(* Logix 5000 AddOnInstructionDefinition export MAH_Yaskawa; software revision 17.00 *)

TYPE Yaskawa_EIP_Servo :   // Yaskawa SigmaLogic Axis Structure v2.4.0
STRUCT
   O : Yaskawa_OUT_to_Servo;
   I : Yaskawa_IN_from_Servo;
   AOI_SB : Yaskawa_AOI_Status_Bits;
END_STRUCT
END_TYPE

TYPE Yaskawa_OUT_to_Servo :   // Structure of data sent out to the Yaskawa SigmaLogic controller v2.4.0
STRUCT
   b00_ServoOn : BOOL;   // Servo On
   b01_Stop : BOOL;   // Stops All Current Motion in Progress
   b02_Home : BOOL;   // Start Homing Process
   b03_MoveStart1 : BOOL;   // Start Current Motion
   b06_SuperImpose : BOOL;
   b07_ServoAlarmReset : BOOL;   // Servo Alarm Reset
   b08_ControllerAlarmReset : BOOL;   // SigmaLogic Alarm Reset
   b09_MoveStart2 : BOOL;   // Start Second Motion (Blended Move)
   b10_MoveAbort : BOOL;   // Abort Current Move
   b11_MovePause : BOOL;   // Pause Current Move
   b12_SeqPause : BOOL;   // Indexing Sequence Pause
   b13_SeqResume : BOOL;   // Indexing Sequence Resume
   b14_SeqCancel : BOOL;   // Indexing Sequence Cancel
   b15_AbsEncoderReset : BOOL;   // Absolute Encoder Reset
   b16_SeqStart : BOOL;   // Start Indexing Sequence
   b17_SeqEditSpeed : BOOL;   // Enter Edit Speed
   b18_SeqEditDistance : BOOL;   // Enter Distance Edit
   b19_PLSEnable : BOOL;   // Enable PLS execution
   b20_PLSActivateOutput1 : BOOL;   // Activate PLS output1 switch logic
   b21_PLSActivateOutput2 : BOOL;   // Activate PLS output2 switch logic
   b22_PLSActivateOutput3 : BOOL;   // Activate PLS output3 switch logic
   b23_PLSActivateOutput4 : BOOL;   // Activate PLS output4 switch logic
   b24_SetClock : BOOL;   // Set the remote controller clock with data provided by the PLC
   RebootController : BOOL;
   UseExternalEncoder : BOOL;   // Use External Encoder when executing MAHSP_Yaskawa
   b32_HeatbeatAnswer : BOOL;   // Heartbeat Answer
   BrakeBypassRequest : BOOL;
   SetFwdTorqueLimit : BOOL;
   SetRevTorqueLimit : BOOL;
   TorqueLimit : DINT;
   TorqueRamp : DINT;
   HomeMethod : INT;
   HomeSpeed : DINT;
   HomeAccDec : DINT;   // Home Move Acceleration/Deceleration Rate
   HomeBackOffDistance : DINT;
   HomeCreepSpeed : DINT;
   HomeCreepDistanceLimit : DINT;
   HomeCreepTimeLimit : DINT;
   HomeOffsetDistance : DINT;
   HomeOffsetSpeed : DINT;
   HomePostion : DINT;
   HomeTorque : DINT;
   HomeInputNo : DINT;
   HomeApproachTimeLimit : DINT;
   HomeApproachDistLimit : DINT;
   HomeDirection : INT;
   HomeSwitchMode : INT;
   MoveType : INT;
   MoveDirection : INT;
   MoveAccel1 : DINT;
   MoveAccel2 : DINT;
   MoveDecel1 : DINT;
   MoveDecel2 : DINT;
   MoveSpeed1 : DINT;
   MoveSpeed2 : DINT;
   MoveDistance1 : DINT;
   MoveDistance2 : DINT;
   MovePosition1 : DINT;
   MovePosition2 : DINT;
   RegistrationDistance : DINT;
   GearNumerator : DINT;
   GearDenominator : DINT;
   SuperImposeDistance : DINT;
   Resolution : INT;
   RegistrationDirection : INT;
   TuningLevel : INT;
   SequenceStep : INT;   // Staring Sequence Step Number
   SequenceEditStep : INT;   // Sequence Step Number to Edit
   FlagCommandBits1 : DINT;   // Flag Commands. 1..64 are General Flags, Bits 0..31 correspond to Flag 1..32
   FlagCommandBits2 : DINT;   // Flag Commands cont. 1..64 are General Flags, Bits 0..31 correspond to Flag 33..64
   DigitalOutCommandBits : DINT;   // Digital Output commands. Bits 0-7 correspond to CN13 Digital Outputs 0-7, used as Flag 73-80. Bits 8-10 correspond to CN1 Digital Outputs 0-2 used as Flag 88-90"
   SequenceEditSpeed : DINT;
   SequenceEditDistance : DINT;
   FeedRateOverride : INT;
   HSI_Enable : BOOL;
   HSI_MoveMode : BOOL;   // 0=Relative; 1=Moves per Cycle
   HSI_CalcMethod : BOOL;   // 0=Accel/Decel; 1=Time
   HSI_MoveDirection : BOOL;   // 0 = Negative; 1 = Positive
   HSI_TriggerFlag : INT;
   HSI_MovingFlag : INT;
   HSI_DwellingFlag : INT;
   HSI_DoneFlag : INT;
   HSI_MoveType : INT;   // 0=Single; 1=Repeat; 2=Repeat "x" times
   HSI_RepeatNumber : INT;
   HSI_Distance : DINT;
   HSI_Speed : DINT;
   HSI_Accel : DINT;
   HSI_MoveTime : DINT;
   HSI_DwellTime : DINT;
   PLS_OutputFlag1 : INT;
   PLS_OutputFlag2 : INT;
   PLS_OutputFlag3 : INT;
   PLS_OutputFlag4 : INT;
   PLS_OnPosition1 : DINT;
   PLS_OffPosition1 : DINT;
   PLS_OnPosition2 : DINT;
   PLS_OffPosition2 : DINT;
   PLS_OnPosition3 : DINT;
   PLS_OffPosition3 : DINT;
   PLS_OnPosition4 : DINT;
   PLS_OffPosition4 : DINT;
   PLS_OnCompensation1 : INT;
   PLS_OffCompensation1 : INT;
   PLS_OnCompensation2 : INT;
   PLS_OffCompensation2 : INT;
   PLS_OnCompensation3 : INT;
   PLS_OffCompensation3 : INT;
   PLS_OnCompensation4 : INT;
   PLS_OffCompensation4 : INT;
   RTC_Year : INT;
   RTC_Month : INT;
   RTC_Day : INT;
   RTC_Hour : INT;
   RTC_Min : INT;
   RTC_Sec : INT;
   StopDecel : DINT;
   AnalogOutput : INT;   // CN13, AO_01 [mV]
END_STRUCT
END_TYPE

TYPE Yaskawa_AOI_Status_Bits :   // Internal bits used to interlock Yaskawa AOI execution. v2.4.0
STRUCT
   MAM : BOOL;   // Move AOI Active
   MAJ : BOOL;   // Jog AOI Active
   MAB : BOOL;   // Blending AOI Active
   MAG : BOOL;   // Gearing AOI Active
   MAHSP : BOOL;   // Home SetPoint AOI Active
   MAH : BOOL;   // Homing AOI Active
   MSQE : BOOL;   // Sequence Edit AOI Active
   MSQR : BOOL;   // Sequence Run AOI Active
   MHSI : BOOL;   // High Speed Index AOI Active
   MSO : BOOL;   // Servo On
   MSF : BOOL;   // Servo Off
   MAFR : BOOL;   // Fault Reset
   MAS : BOOL;   // Servo Abort
   MTRQ : BOOL;   // Torque Mode Active
   MPLS : BOOL;   // PLS Active
   MCLK : BOOL;   // SetClock Active
   MSTL : BOOL;   // Set Torque Limit Active
   AOI_Permissive : BOOL;   // Permissive to Execute an AOI
END_STRUCT
END_TYPE

TYPE Yaskawa_IN_from_Servo :   // Structure of data coming from the Yaskawa SigmaLogic controller. v2.4.0
STRUCT
   AlarmText : STRING;   // ServoPack Alarm Code plus Text Description
   b00_Heartbeat : BOOL;
   b01_Alarm : BOOL;   // ServoPack Alarm
   b02_Warning : BOOL;   // ServoPack Warning
   b03_Ready : BOOL;   // ServoPack Ready
   b04_Enabled : BOOL;   // ServoPack Enabled ("Servo On")
   b05_StopComplete : BOOL;
   b06_HomeComplete : BOOL;
   b07_HomeBusy : BOOL;
   b08_HomeActive : BOOL;
   b09_HomeAborted : BOOL;
   b10_HomeError : BOOL;
   b11_MoveAbsComplete : BOOL;
   b12_MoveAbsBusy : BOOL;
   b13_MoveAbsActive : BOOL;
   b14_MoveAbsAborted : BOOL;
   b15_MoveAbsError : BOOL;
   b16_MoveRelComplete : BOOL;
   b17_MoveRelBusy : BOOL;
   b18_MoveRelActive : BOOL;
   b19_MoveRelAborted : BOOL;
   b20_MoveRelError : BOOL;
   b21_JogAtSpeed : BOOL;
   b22_JogBusy : BOOL;
   b23_JogActive : BOOL;
   b24_JogAborted : BOOL;
   b25_JogError : BOOL;
   b26_GearInSync : BOOL;
   b27_GearBusy : BOOL;
   b28_GearActive : BOOL;
   b29_GearAborted : BOOL;
   b30_GearError : BOOL;
   b32_MoveSuperComplete : BOOL;
   b33_MoveSuperBusy : BOOL;
   b34_MoveSuperActive : BOOL;
   b35_MoveSuperAborted : BOOL;
   b36_MoveSuperError : BOOL;
   b37_PowerCycleRequired : BOOL;
   b38_MoveBlend1Complete : BOOL;
   b39_MoveBlend1Busy : BOOL;
   b40_MoveBlend1Active : BOOL;
   b41_MoveBlend1Abort : BOOL;
   b42_MoveBlend1Error : BOOL;
   b43_MoveBlend2Complete : BOOL;
   b44_MoveBlend2Busy : BOOL;
   b45_MoveBlend2Active : BOOL;
   b46_MoveBlend2Abort : BOOL;
   b47_MoveBlend2Error : BOOL;
   b48_RegComplete : BOOL;
   b49_RegBusy : BOOL;
   b50_RegActive : BOOL;
   b51_RegAborted : BOOL;
   b52_RegError : BOOL;
   b53_ResetAbsEncoderActive : BOOL;
   b54_ResetAbsEncoderBusy : BOOL;
   b55_ResetAbsEncoderDone : BOOL;
   b56_ResetAbsEncoderError : BOOL;
   b57_SeqRunning : BOOL;
   b58_RegSensorNotReached : BOOL;
   b59_SeqEditError : BOOL;
   b60_SeqEditDone : BOOL;
   b61_TorqueAtTorque : BOOL;
   b62_TorqueBusy : BOOL;
   b63_TorqueActive : BOOL;
   b64_TorqueAborted : BOOL;
   b65_TorqueError : BOOL;
   b66_ControllerAlarm : BOOL;
   b67_ApplicationError : BOOL;
   b68_AxisAtStandStill : BOOL;
   b69_TestModeActive : BOOL;
   b70_ServoParamsOK : BOOL;
   b71_SetFwdTorqueLimitDone : BOOL;
   b72_SetRevTorqueLimitDone : BOOL;
   Position : DINT;
   Speed : DINT;
   Torque : DINT;
   HomeErrorID : INT;
   MoveAbsErrorID : INT;
   MoveRelErrorID : INT;
   JogErrorID : INT;
   GearErrorID : INT;
   MoveSuperErrorID : INT;
   ServoAlarmID : INT;
   ServoWarningID : INT;
   ControllerAlarmID : DINT;
   AxisGenAlarmID : DINT;
   MoveBlend1ErrorID : INT;
   MoveBlend2ErrorID : INT;
   ResetAbsEncoderErrorID : INT;
   FunctionBlockErrorID : INT;
   TorqueErrorID : INT;
   RegErrorID : INT;
   SeqCurrentStep : INT;
   FlagStatusBit1 : DINT;   // Flag Status. 1..64 are General Flags, Bits 0..31 correspond to Flag 1..32
   FlagStatusBit2 : DINT;   // Flag Status cont. 1..64 are General Flags, Bits 0..31 correspond to Flag 33..64
   IOStatusBits : DINT;   // Digital IO Status. Bits 0-7, CN13 Inputs 0-7, Used as Flag 65-72. Bits 8-15, CN13 Outputs 0-7, Used as Flag 73-80. Bits 16-22, CN1 Inputs 0-6, Used as Flag 81-87. Bits 23-25, CN1 Outputs 0-4, Used as Flag 88-92.
   HSI_Moving : BOOL;
   HSI_Dwelling : BOOL;
   HSI_Done : BOOL;
   HSI_Busy : BOOL;
   HSI_Error : BOOL;
   HSI_ErrorCode : INT;
   PLS_Running : BOOL;
   PLS_SwitchStatus1 : BOOL;
   PLS_SwitchStatus2 : BOOL;
   PLS_SwitchStatus3 : BOOL;
   PLS_SwitchStatus4 : BOOL;
   PLS_Busy : BOOL;
   PLS_Error : BOOL;
   PLS_ErrorCode : INT;
   SetClock_Done : BOOL;
   SetClock_Busy : BOOL;
   SetClock_Error : BOOL;
   SetClock_ErrorID : INT;
   SoftwareVersion : DINT;
   FirmwareVersion : DINT;
   CommandedPos : DINT;
   CommandedPosNonCyc : DINT;
   CommandedSpeed : DINT;
   Clock_Year : INT;
   Clock_Month : INT;
   Clock_Day : INT;
   Clock_Hour : INT;
   Clock_Minute : INT;
   Clock_Second : INT;
   AnalogInput : REAL;   // CN13, AI_01 [v]
   BrakeBypassActive : BOOL;
   ForwardTorqueLimit : DINT;
   ReverseTorqueLimit : DINT;
END_STRUCT
END_TYPE

ADD_ON_INSTRUCTION MAH_Yaskawa   (* revision 2.4 0, vendor Yaskawa America, Inc., ExecuteEnableInFalse *)
// Motion Axis Home
// Revision note:
// 2.4.0: Improved Error Codes for invalid homing parameters.
// 2.3.1: Moved unlatch of AOI_ON_LOCAL to bottom of EnableInFalse routine so that outputs will be on for at least 1 scan if one-shot on EN is used.
// 2.3.0: No functional change
// 2.0.0: Added new Homing type for C-Pulse Only (Type 4), The ORDER OF THE INPUTS HAS CHANGED. Check attached tags for existing projects!
// Help:
// This AOI moves a servo axis to a home position by various methods. Timeouts are not directly included in this AOI and should be implemented in user code. Supported Homing Methods include:
// - Set Position Only
// - To Hard Stop.
// - To Overtravel (P-OT, N-OT) w/wo encoder C-Channel
// - To Flag w/wo encoder C-Channel (Flag can also be one of the Controller Digital Inputs)
//     CN1 Inputs: SI0...SI6 = Flag 81...Flag 87
//     CN13 Inputs: DI_00... DI_07 = Flag 65...Flag72
// 'Set Position Only' can occur whether the servo is enabled or disabled. Position will be immediately set to the specified value.
// Home to Hard Stop moves the servo under a Torque Limit until the hard stop is reached according to the following sequence:
// - Backoff move is always performed in the opposite direction of the search Direction. Always use a Positive Value for BackoffDistance
// - TorqueLimit is set and the axis moves to the hard stop in the specified Direction under max Speed limit.
// - When hard stop is reached, Offset move is performed according to the value set in OffsetDistance and OffsetSpeed. Direction will always be opposite to the searching direction.
// - Position is defined as the SetPosition
// Home to Overtravel (P-OT, N-OT) or Flag without C-Channel performs the following sequence:
// - Initial search (Approach) in specified Direction.
// - TorqueLimit is active
// - When Overtravel switch or Flag is found,  move the BackoffDistance. Always use a Positive Value for BackoffDistance. Direction will be automatically opposite of search direction
// - Final search is performed (Creep) in the specified Direction using CreepSpeed
// - When Overtravel switch or Flag is found again,  Offset move is performed according to the value set in OffsetDistance and OffsetSpeed. Direction will be automatically opposite of serach direction.
// - Position is defined as the SetPosition
// Home to Overtravel (P-OT, N-OT) or Flag with C-Channel performs the following sequence:
// - Initial search (Approach) in specified Direction.
// - TorqueLimit is active
// - When Overtravel switch or Flag is found,  move the BackoffDistance. Always use a Positive Value for BackoffDistance. Direction will be automatically opposite of search direction
// - Final search is performed (Creep) in the specified Direction using CreepSpeed
// - When C-Channel is found,  Offset move is performed according to the value set in OffsetDistance and OffsetSpeed. Direction will be automatically opposite of serach direction.
// - Position is defined as the SetPosition
// Error Codes:
// 13017: Invalid Homing Parameters
// 13018: Invalid Move Type - Overtravel(s) are disabled
// 13019: Home Input not found
// 13020: Invalid Homing Type
// 13021: Invalid Accel/Decel Parameter
// 13022: Invalid Velocity Parameter
// 13023: Invalid Torque Parameter
// 13024: Invalid Position Parameter
VAR_IN_OUT
   Axis : Yaskawa_EIP_Servo; {required}
END_VAR
VAR_INPUT
   HomeType : INT := 1; {required}   // 0 = Set Position 1 = Home to Hard Stop 2 = Home to Overtravel Switch 3 = Home to Flag 4= Home to C-Pulse Only
   Direction : INT; {required}   // 0 = Positive 1 = Negative
   Use_CPulse : INT; {required}   // 0 = Do Not Use C-Pulse 1 = Use C-Pulse
   Accel_Decel : REAL; {required}   // Homing Accel/Decel [unit/s/s]
   Speed : REAL; {required}   // Homing Speed [unit/s]
   TorqueLimit : REAL; {required}   // Torque or Force Limit for Homing [%motor rated torque/force]
   FlagNo : INT; {required}   // SigmaLogic Flag to use as Trigger for Home Type 3
   BackoffDistance : REAL; {required}   // Distance to back off before moving to hard stop (Type 1) or after finding the overtravel or flag (Types 2 and 3)
   CreepSpeed : REAL; {required}   // Homing Creep Speed [units/s]
   OffsetDistance : REAL; {required}   // Homing Offset Distance [unit]
   OffsetSpeed : REAL; {required}   // Homing Offset Speed [unit/s]
   SetPosition : REAL; {required}   // Position to Define at end of homing process
   ApproachDistanceLimit : REAL;   // (Not supported)
   ApproachTimeLimit : REAL;   // (Not supported)
   CreepDistLimit : REAL;   // (Not supported)
   CreepTimeLimit : REAL;   // (Not supported)
END_VAR
VAR_OUTPUT
   EN : BOOL; {visible}   // The AOI is Active
   DN : BOOL; {visible}   // Homing is Done
   IP : BOOL; {visible}   // Homing is In Process
   ER : BOOL; {visible}   // Homing Process Error
   PC : BOOL; {visible}   // Homing Process is Successfully Completed
   FLT_RDY : BOOL; {visible}   // The Servo is Not Ready
   FLT_BSY : BOOL; {visible}   // There is another AOI Active for this Axis
   ErrorCode : INT; {visible}   // Homing process Error Code
END_VAR
VAR
   AOI_ON_LOCAL : BOOL;
   ScaleFactor : DINT;
   Finished : BOOL;   // Function is finished
   Execute_OS : BOOL;
END_VAR

ROUTINE EnableInFalse   (* ladder *)
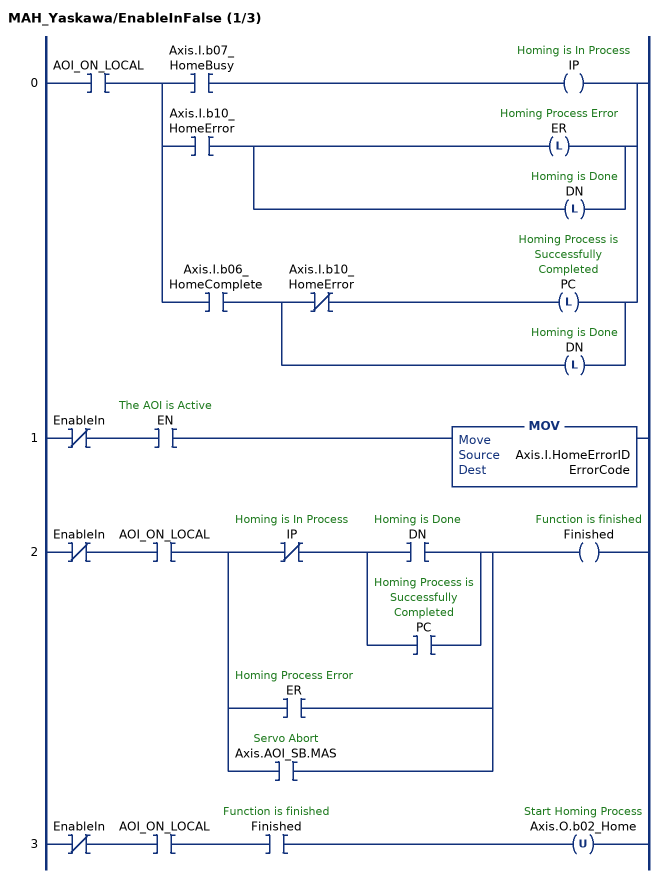
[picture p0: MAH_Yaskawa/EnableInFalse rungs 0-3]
   0: XIC(AOI_ON_LOCAL)[XIC(Axis.I.b07_HomeBusy) OTE(IP) ,XIC(Axis.I.b10_HomeError) [OTL(ER) ,OTL(DN) ] ,XIC(Axis.I.b06_HomeComplete) [XIO(Axis.I.b10_HomeError) OTL(PC) ,OTL(DN) ] ];
   1: XIO(EnableIn)XIC(EN)MOV(Axis.I.HomeErrorID,ErrorCode);
   2: XIO(EnableIn)XIC(AOI_ON_LOCAL)[XIO(IP) [XIC(DN) ,XIC(PC) ] ,XIC(ER) ,XIC(Axis.AOI_SB.MAS) ]OTE(Finished);
   3: XIO(EnableIn)XIC(AOI_ON_LOCAL)XIC(Finished)OTU(Axis.O.b02_Home);
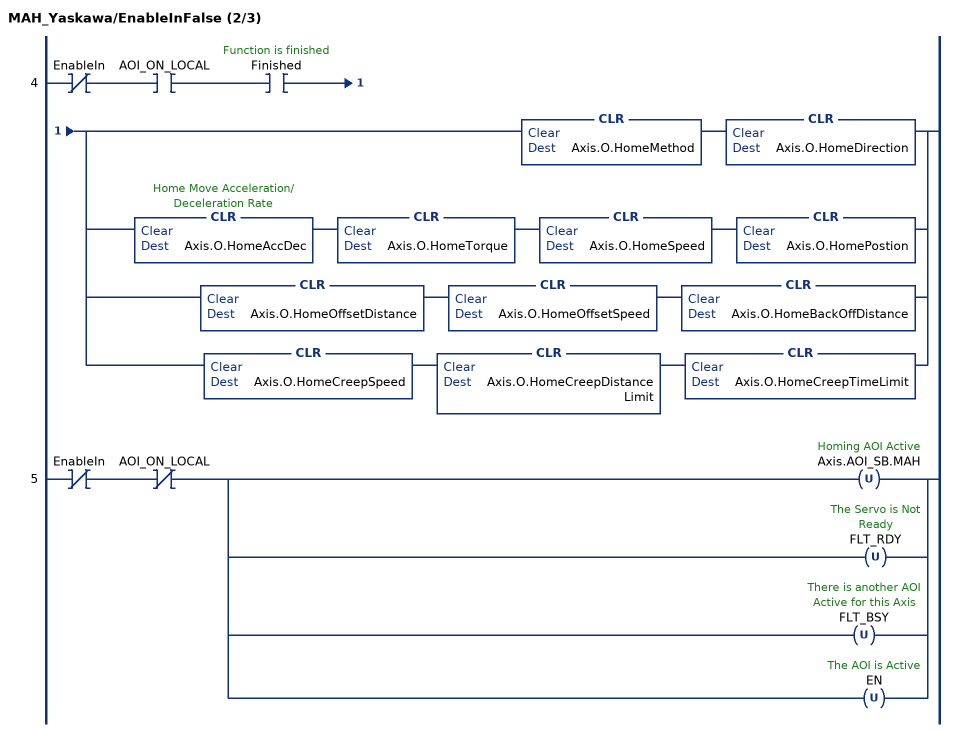
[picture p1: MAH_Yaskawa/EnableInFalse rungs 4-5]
   4: XIO(EnableIn)XIC(AOI_ON_LOCAL)XIC(Finished)[CLR(Axis.O.HomeMethod) CLR(Axis.O.HomeDirection) ,CLR(Axis.O.HomeAccDec) CLR(Axis.O.HomeTorque) CLR(Axis.O.HomeSpeed) CLR(Axis.O.HomePostion) ,CLR(Axis.O.HomeOffsetDistance) CLR(Axis.O.HomeOffsetSpeed) CLR(Axis.O.HomeBackOffDistance) ,CLR(Axis.O.HomeCreepSpeed) CLR(Axis.O.HomeCreepDistanceLimit) CLR(Axis.O.HomeCreepTimeLimit) ];
   5: XIO(EnableIn)XIO(AOI_ON_LOCAL)[OTU(Axis.AOI_SB.MAH) ,OTU(FLT_RDY) ,OTU(FLT_BSY) ,OTU(EN) ];
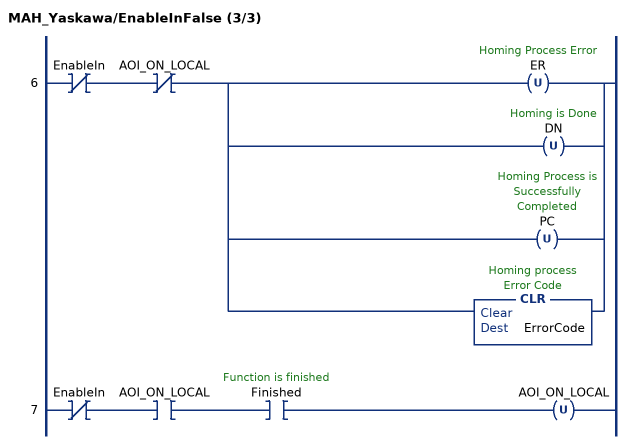
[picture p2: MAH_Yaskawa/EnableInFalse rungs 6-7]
   6: XIO(EnableIn)XIO(AOI_ON_LOCAL)[OTU(ER) ,OTU(DN) ,OTU(PC) ,CLR(ErrorCode) ];
   7: XIO(EnableIn)XIC(AOI_ON_LOCAL)XIC(Finished)OTU(AOI_ON_LOCAL);
END_ROUTINE

ROUTINE Logic   (* ladder *)
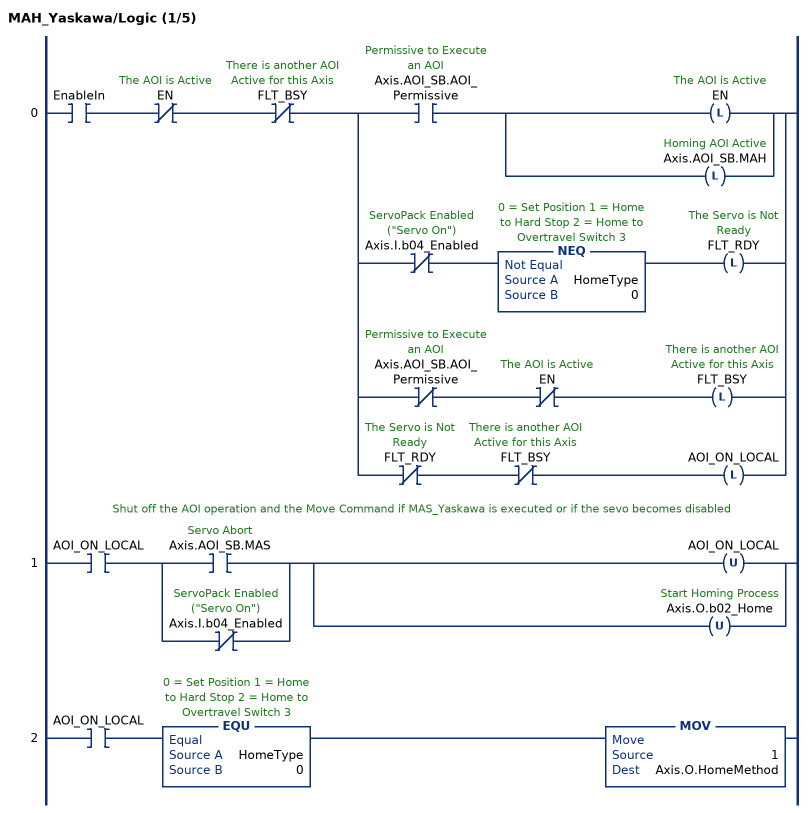
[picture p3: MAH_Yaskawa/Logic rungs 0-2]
   0: XIC(EnableIn)XIO(EN)XIO(FLT_BSY)[XIC(Axis.AOI_SB.AOI_Permissive) [OTL(EN) ,OTL(Axis.AOI_SB.MAH) ] ,XIO(Axis.I.b04_Enabled) NEQ(HomeType,0) OTL(FLT_RDY) ,XIO(Axis.AOI_SB.AOI_Permissive) XIO(EN) OTL(FLT_BSY) ,XIO(FLT_RDY) XIO(FLT_BSY) OTL(AOI_ON_LOCAL) ];
   // Shut off the AOI operation and the Move Command if MAS_Yaskawa is executed or if the sevo becomes disabled
   1: XIC(AOI_ON_LOCAL)[XIC(Axis.AOI_SB.MAS) ,XIO(Axis.I.b04_Enabled) ][OTU(AOI_ON_LOCAL) ,OTU(Axis.O.b02_Home) ];
   2: XIC(AOI_ON_LOCAL)EQU(HomeType,0)MOV(1,Axis.O.HomeMethod);
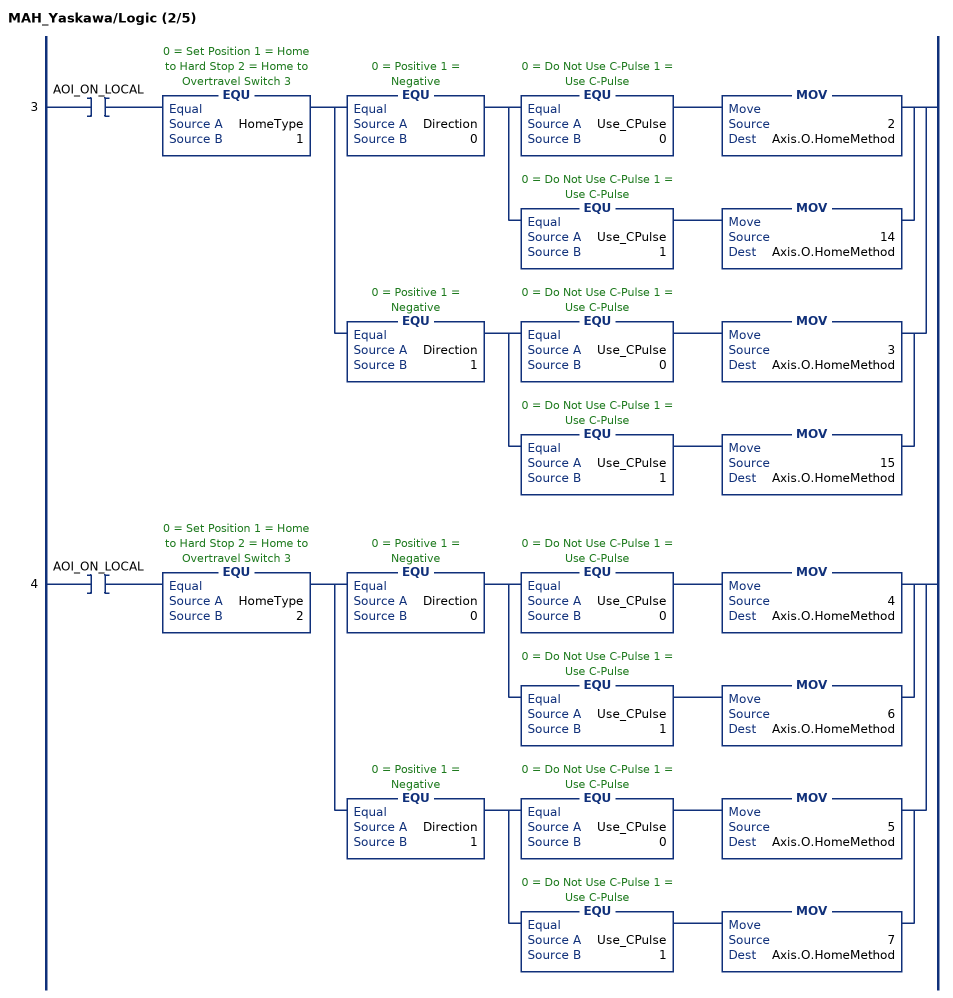
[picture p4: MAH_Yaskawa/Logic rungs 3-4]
   3: XIC(AOI_ON_LOCAL)EQU(HomeType,1)[EQU(Direction,0) [EQU(Use_CPulse,0) MOV(2,Axis.O.HomeMethod) ,EQU(Use_CPulse,1) MOV(14,Axis.O.HomeMethod) ] ,EQU(Direction,1) [EQU(Use_CPulse,0) MOV(3,Axis.O.HomeMethod) ,EQU(Use_CPulse,1) MOV(15,Axis.O.HomeMethod) ] ];
   4: XIC(AOI_ON_LOCAL)EQU(HomeType,2)[EQU(Direction,0) [EQU(Use_CPulse,0) MOV(4,Axis.O.HomeMethod) ,EQU(Use_CPulse,1) MOV(6,Axis.O.HomeMethod) ] ,EQU(Direction,1) [EQU(Use_CPulse,0) MOV(5,Axis.O.HomeMethod) ,EQU(Use_CPulse,1) MOV(7,Axis.O.HomeMethod) ] ];
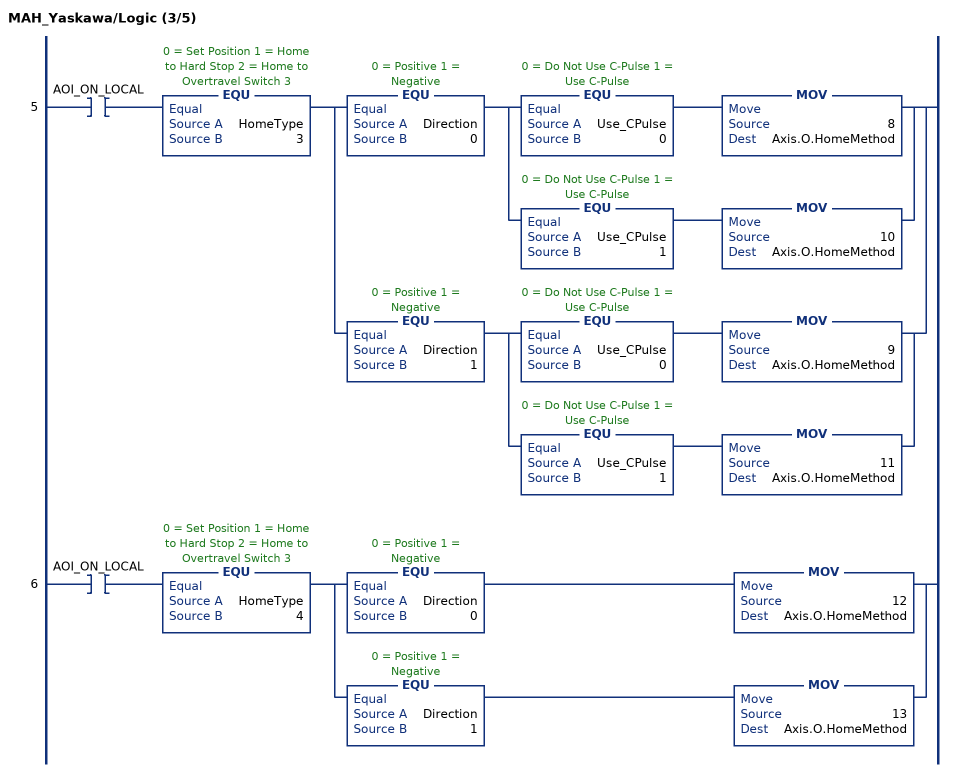
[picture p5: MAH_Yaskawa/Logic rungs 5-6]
   5: XIC(AOI_ON_LOCAL)EQU(HomeType,3)[EQU(Direction,0) [EQU(Use_CPulse,0) MOV(8,Axis.O.HomeMethod) ,EQU(Use_CPulse,1) MOV(10,Axis.O.HomeMethod) ] ,EQU(Direction,1) [EQU(Use_CPulse,0) MOV(9,Axis.O.HomeMethod) ,EQU(Use_CPulse,1) MOV(11,Axis.O.HomeMethod) ] ];
   6: XIC(AOI_ON_LOCAL)EQU(HomeType,4)[EQU(Direction,0) MOV(12,Axis.O.HomeMethod) ,EQU(Direction,1) MOV(13,Axis.O.HomeMethod) ];
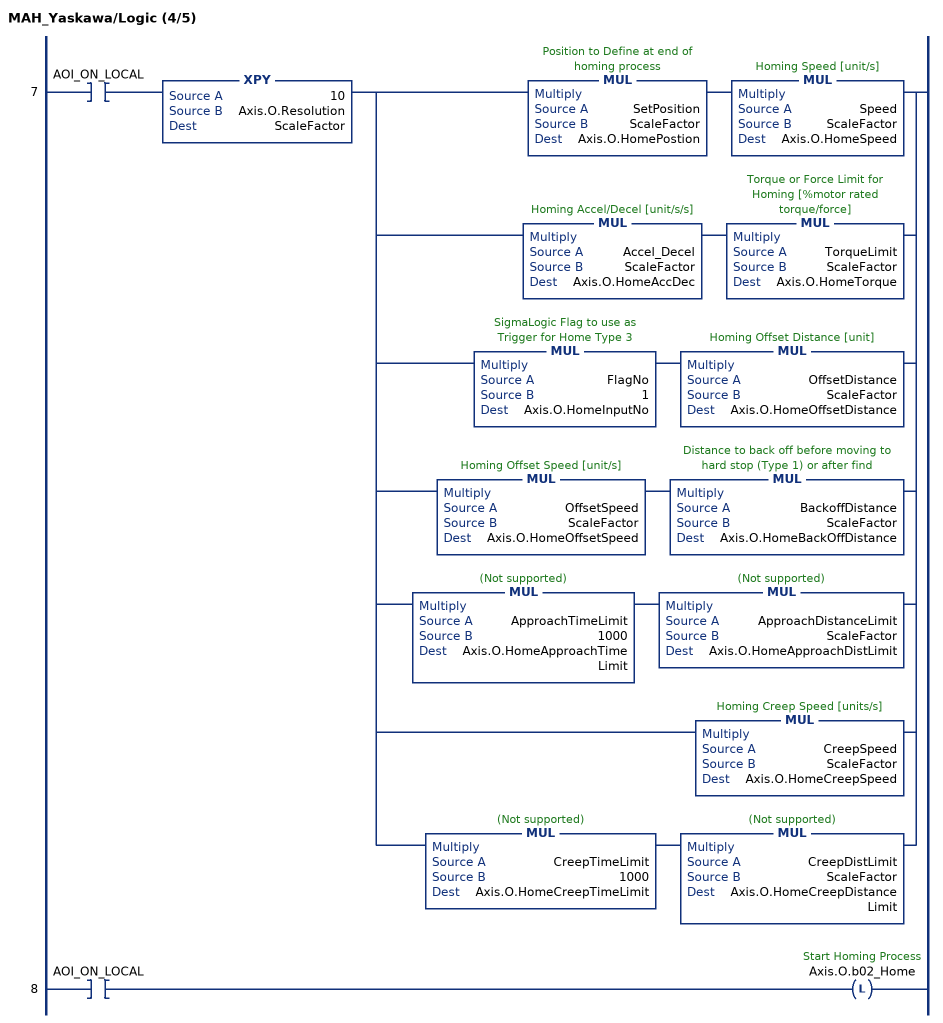
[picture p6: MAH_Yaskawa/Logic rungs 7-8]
   7: XIC(AOI_ON_LOCAL)XPY(10,Axis.O.Resolution,ScaleFactor)[MUL(SetPosition,ScaleFactor,Axis.O.HomePostion) MUL(Speed,ScaleFactor,Axis.O.HomeSpeed) ,MUL(Accel_Decel,ScaleFactor,Axis.O.HomeAccDec) MUL(TorqueLimit,ScaleFactor,Axis.O.HomeTorque) ,MUL(FlagNo,1,Axis.O.HomeInputNo) MUL(OffsetDistance,ScaleFactor,Axis.O.HomeOffsetDistance) ,MUL(OffsetSpeed,ScaleFactor,Axis.O.HomeOffsetSpeed) MUL(BackoffDistance,ScaleFactor,Axis.O.HomeBackOffDistance) ,MUL(ApproachTimeLimit,1000,Axis.O.HomeApproachTimeLimit) MUL(ApproachDistanceLimit,ScaleFactor,Axis.O.HomeApproachDistLimit) ,MUL(CreepSpeed,ScaleFactor,Axis.O.HomeCreepSpeed) ,MUL(CreepTimeLimit,1000,Axis.O.HomeCreepTimeLimit) MUL(CreepDistLimit,ScaleFactor,Axis.O.HomeCreepDistanceLimit) ];
   8: XIC(AOI_ON_LOCAL)OTL(Axis.O.b02_Home);
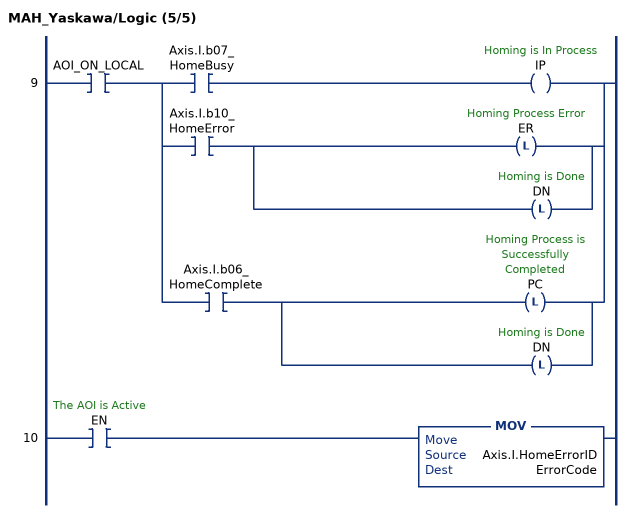
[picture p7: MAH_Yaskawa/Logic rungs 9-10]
   9: XIC(AOI_ON_LOCAL)[XIC(Axis.I.b07_HomeBusy) OTE(IP) ,XIC(Axis.I.b10_HomeError) [OTL(ER) ,OTL(DN) ] ,XIC(Axis.I.b06_HomeComplete) [OTL(PC) ,OTL(DN) ] ];
   10: XIC(EN)MOV(Axis.I.HomeErrorID,ErrorCode);
END_ROUTINE
END_ADD_ON_INSTRUCTION
